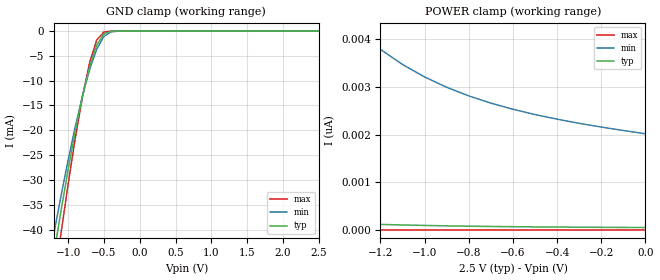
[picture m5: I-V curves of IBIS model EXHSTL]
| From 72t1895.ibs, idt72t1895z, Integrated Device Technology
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|   Model EXHSTL
[Model]   EXHSTL
Model_type   Input
Vinl =  0.400V
Vinh =  1.400V
Vmeas =  0.900V
C_comp   3.00pF   NA   NA
[Temperature Range]   25.00   85.00   -40.00
[Voltage Range]   2.50V   2.30V   2.70V
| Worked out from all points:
|   GND clamp passes 1 mA (typ) near -0.52 V on its own axis
[GND_clamp]
| voltage   I(typ)   I(min)   I(max)
-2.5V     -171mA     -153mA     -195mA
-1.2V     -45.09mA   -40.91mA   -51.2mA
-1.1V     -36.28mA   -33.25mA   -40.8mA
-1V       -27.91mA   -25.98mA   -30.84mA
-900mV    -20.11mA   -19.21mA   -21.55mA
-800mV    -13.1mA    -13.07mA   -13.22mA
-700mV    -7.177mA   -7.773mA   -6.35mA
-600mV    -2.805mA   -3.616mA   -1.783mA
-500mV    -571uA     -1.059mA   -188uA
-400mV    -51.63uA   -157uA     -8.189uA
-300mV    -2.312uA   -13.07uA   -119nA
2.5V      50.98pA    2.159nA    204fA
[POWER_clamp]
| voltage   I(typ)   I(min)   I(max)
-2.5V     750pA      20.77nA    2.711pA
-2.3V     558pA      15.53nA    2.052pA
-2V       355pA      10.06nA    1.341pA
-1.7V     228pA      6.656nA    893fA
-1.3V     132pA      4.17nA     553fA
-1.2V     117pA      3.787nA    493fA
-1.1V     105pA      3.471nA    451fA
-1V       94.88pA    3.209nA    410fA
-800mV    79.45pA    2.812nA    350fA
-500mV    64.69pA    2.421nA    286fA
-300mV    58.18pA    2.237nA    256fA
0V        50.98pA    2.018nA    221fA
